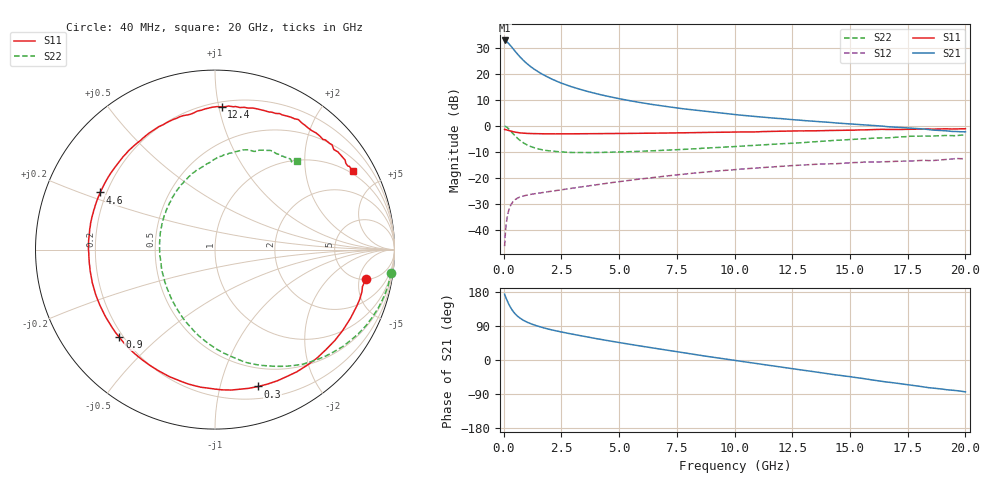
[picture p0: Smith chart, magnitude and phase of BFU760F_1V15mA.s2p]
! Filename:  P:\Prog\Test\Noise\ATS_data\Testdata_Net\Split files Spar\BFU760F_2W_C1_1V_5mA_60mA_Bias4_D.s2p
! Date/Time: Mon 06/Feb/2012 15:06:07
! BFU760_2W_C1_1V_5mA_60mA_Bias4_R.s2p
! MDIF S-parameter v. bias file
! BFU760_2W_C1_1V_5mA_60mA
! Date/time Fri Mar 18 10:56:44 2011
! VAR V_out= 1.0001
! VAR I_out= 14.9950
! VAR V_in= 0.7871
! VAR I_in= 0.0452
! Device data file deembeded for feedlines and parallel
! Original file: \Split files Spar\BFU760_2W_C1_1V_5mA_60mA_Bias4_R.s2p
! Feed-files: PR003V01_101208_Feed1.s2p, PR003V01_101208_Feed2.s2p
! Parallel-file: PR003V01_101208_Par.s2p
# MHz S MA R 50
!  Freq-MHz  S11-mag  S11-arg  S21-mag  S21-arg  S12-mag  S12-arg  S22-mag  S22-arg
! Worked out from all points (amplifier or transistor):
!   167 points, 40 MHz to 20 GHz, reference 50 ohm
!   highest |S21| = 32.8 dB at 40 MHz (marker M1)
!   |S21| within 3 dB of that: start of sweep to 392.5 MHz
!   unconditionally stable (mu >= 1): 4.668 GHz to 15 GHz
!   at 550 MHz: K = 0.19, MSG = 28.0 dB, |S12| = -28.0 dB
!   at 4.2 GHz: K = 0.97, MSG = 17.2 dB, |S12| = -22.4 dB
!   at 20 GHz: K = 0.91, MSG = 5.1 dB, |S12| = -12.6 dB
!   S11 on the Smith chart (normalised r, x): 40 MHz: 5.12, -6.27; 300 MHz: 0.31, -1.32; 900 MHz: 0.18, -0.38; 4.6 GHz: 0.18, +0.23; 12.4 GHz: 0.23, +1.02; 20 GHz: 0.90, +3.57
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40  0.8563 -11.0  43.69 173.7  0.004923 84.3  0.9893 -7.6
50  0.847 -14.1  43.56 171.5  0.005956 79.3  0.9868 -9.7
90  0.8471 -24.5  42.7 165.4  0.01091 78.0  0.9721 -17.4
160  0.8322 -42.1  40.19 155.2  0.0185 69.3  0.9259 -30.5
240  0.8124 -60.6  37.25 144.9  0.02559 60.8  0.8566 -43.7
300  0.7999 -72.5  34.45 138.4  0.0298 55.4  0.8034 -52.7
400  0.7771 -90.1  30.64 129.0  0.03504 48.3  0.7131 -65.3
480  0.7636 -101.2  27.58 123.1  0.03805 43.8  0.655 -74.2
550  0.7521 -109.7  25.37 118.5  0.03993 40.8  0.6057 -80.8
700  0.7357 -123.8  21.26 110.9  0.04313 36.1  0.5304 -93.0
900  0.723 -137.4  17.32 103.3  0.0459 32.5  0.4602 -106.0
1300  0.7119 -154.9  12.48 92.9  0.04971 29.3  0.3837 -125.3
1850  0.7059 -169.5  8.921 82.9  0.05402 28.5  0.338 -143.7
2500  0.7054 178.9  6.629 73.9  0.05938 29.2  0.318 -159.0
3400  0.7084 166.9  4.906 63.2  0.06798 29.4  0.3091 -174.1
4600  0.7147 153.6  3.627 50.2  0.08079 28.5  0.3124 169.9
6800  0.7289 132.9  2.445 28.5  0.1063 22.4  0.3385 147.0
10200  0.766 104.7  1.621 -2.9  0.1471 6.5  0.4085 117.2
12400  0.796 87.4  1.337 -22.0  0.1723 -5.8  0.4632 99.6
13400  0.8034 80.1  1.231 -30.5  0.1829 -12.8  0.493 92.3
16800  0.8551 54.1  0.9549 -59.5  0.2073 -33.8  0.5963 66.8
20000  0.8824 29.6  0.7698 -84.1  0.2352 -55.0  0.6703 47.2
